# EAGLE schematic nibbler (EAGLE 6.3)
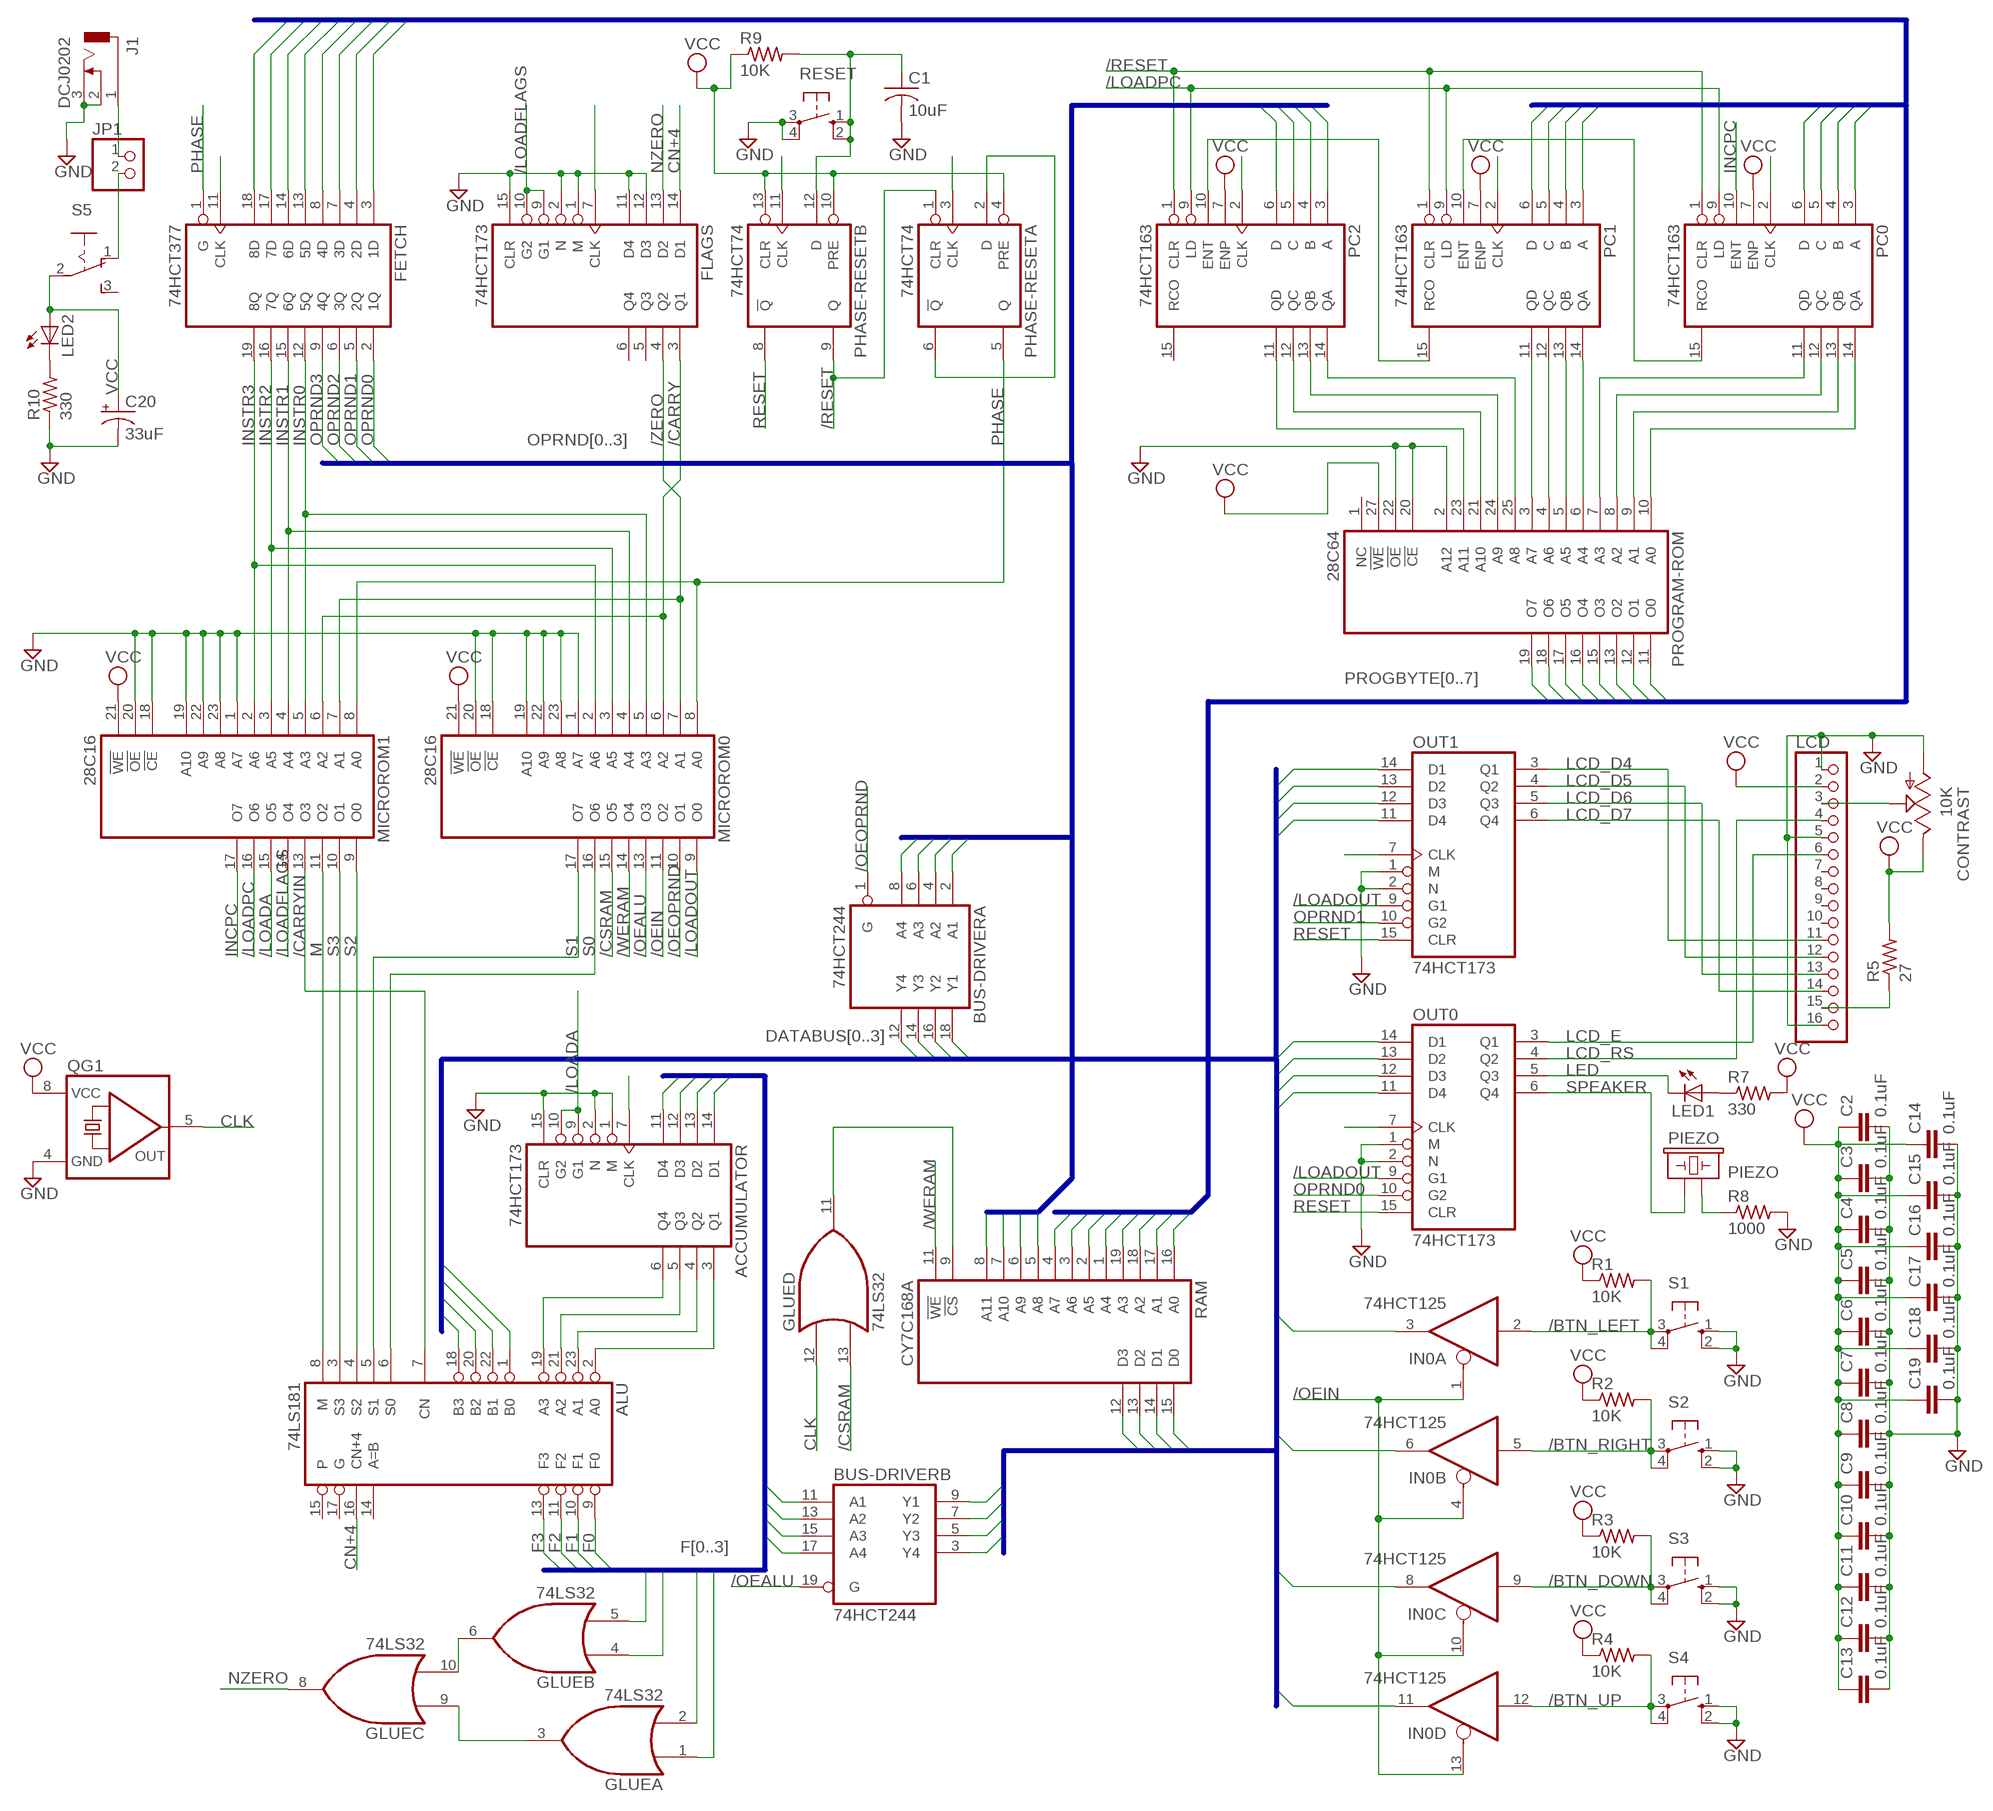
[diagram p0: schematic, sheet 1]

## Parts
ACCUMULATOR  74HCT173  74LS173N  [DIL16]
ALU  74LS181  74LS181N  [DIL24-6]
BUS-DRIVER  74HCT244  74LS244N  [DIL20]
C1  10uF  C-US025-024X044  [C025-024X044]
C2  0.1uF  C2,5-3  [C2.5-3]
C3  0.1uF  C2,5-3  [C2.5-3]
C4  0.1uF  C2,5-3  [C2.5-3]
C5  0.1uF  C2,5-3  [C2.5-3]
C6  0.1uF  C2,5-3  [C2.5-3]
C7  0.1uF  C2,5-3  [C2.5-3]
C8  0.1uF  C2,5-3  [C2.5-3]
C9  0.1uF  C2,5-3  [C2.5-3]
C10  0.1uF  C2,5-3  [C2.5-3]
C11  0.1uF  C2,5-3  [C2.5-3]
C12  0.1uF  C2,5-3  [C2.5-3]
C13  0.1uF  C2,5-3  [C2.5-3]
C14  0.1uF  C2,5-3  [C2.5-3]
C15  0.1uF  C2,5-3  [C2.5-3]
C16  0.1uF  C2,5-3  [C2.5-3]
C17  0.1uF  C2,5-3  [C2.5-3]
C18  0.1uF  C2,5-3  [C2.5-3]
C19  0.1uF  C2,5-3  [C2.5-3]
C20  33uF  CPOL-USTT5D10  [TT5D10]
CONTRAST  10K  TRIM_US-B25P  [B25P]
FETCH  74HCT377  74LS377N  [DIL20]
FLAGS  74HCT173  74LS173N  [DIL16]
GLUE  74LS32  74*32N  [DIL14]
IN0  74HCT125  74125N  [DIL14]
J1  DCJ0202  [DCJ0202]
JP1  PINHD-1X2  [1X02]
LCD  PINHD-1X16  [1X16]
LED1  LED5MM  [LED5MM]
LED2  LED5MM  [LED5MM]
MICROROM0  28C16  [DIL24]
MICROROM1  28C16  [DIL24]
OUT0  74HCT173  74LS173N  [DIL16]
OUT1  74HCT173  74LS173N  [DIL16]
PC0  74HCT163  74163N  [DIL16]
PC1  74HCT163  74163N  [DIL16]
PC2  74HCT163  74163N  [DIL16]
PHASE-RESET  74HCT74  74LS74N  [DIL14]
PIEZO  PIEZO  [PIEZO-12.6MM]
PROGRAM-ROM  28C64  [DIL28]
QG1  QG5460  [DIL08S]
R1  10K  R-US_0204/5  [0204/5]
R2  10K  R-US_0204/5  [0204/5]
R3  10K  R-US_0204/5  [0204/5]
R4  10K  R-US_0204/5  [0204/5]
R5  27  R-US_0204/5  [0204/5]
R7  330  R-US_0204/5  [0204/5]
R8  1000  R-US_0204/5  [0204/5]
R9  10K  R-US_0204/5  [0204/5]
R10  330  R-US_0204/5  [0204/5]
RAM  CY7C168A  51C68  [DIL20]
RESET  10-XX  [B3F-10XX]
S1  10-XX  [B3F-10XX]
S2  10-XX  [B3F-10XX]
S3  10-XX  [B3F-10XX]
S4  10-XX  [B3F-10XX]
S5  255SB  [255SB]

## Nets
/BTN_DOWN: IN0.9(C:I) R3.2 S3.3(P) S3.4(P1)
/BTN_LEFT: IN0.2(A:I) R1.2 S1.3(P) S1.4(P1)
/BTN_RIGHT: IN0.5(B:I) R2.2 S2.3(P) S2.4(P1)
/BTN_UP: IN0.12(D:I) R4.2 S4.3(P) S4.4(P1)
/CARRY: FLAGS.3(Q1) MICROROM0.6(A2) MICROROM1.6(A2)
/CARRYIN: ALU.7(CN) MICROROM1.13(O3)
/CSRAM: GLUE.13(D:I1) MICROROM0.15(O5)
/LOADA: ACCUMULATOR.9(G1) ACCUMULATOR.10(G2) MICROROM1.15(O5)
/LOADFLAGS: FLAGS.9(G1) FLAGS.10(G2) MICROROM1.14(O4)
/LOADOUT: MICROROM0.9(O0) OUT0.9(G1) OUT1.9(G1)
/LOADPC: MICROROM1.16(O6) PC0.9(LD) PC1.9(LD) PC2.9(LD)
/OEALU: BUS-DRIVER.19(B:G) MICROROM0.13(O3)
/OEIN: IN0.1(A:OE) IN0.4(B:OE) IN0.10(C:OE) IN0.13(D:OE) MICROROM0.11(O2)
/OEOPRND: BUS-DRIVER.1(A:G) MICROROM0.10(O1)
/RESET: PC0.1(CLR) PC1.1(CLR) PC2.1(CLR) PHASE-RESET.1(A:CLR) PHASE-RESET.9(B:Q)
/WERAM: MICROROM0.14(O4) RAM.11(!WE)
/ZERO: FLAGS.4(Q2) MICROROM0.7(A1) MICROROM1.7(A1)
CLK: ACCUMULATOR.7(CLK) FETCH.11(CLK) FLAGS.7(CLK) GLUE.12(D:I0) OUT0.7(CLK) OUT1.7(CLK) PC0.2(CLK) PC1.2(CLK) PC2.2(CLK) PHASE-RESET.3(A:CLK) PHASE-RESET.11(B:CLK) QG1.5(OUT)
CN+4: ALU.16(CN+4) FLAGS.14(D1)
DATABUS0: ALU.1(B0) BUS-DRIVER.9(B:Y1) BUS-DRIVER.18(A:Y1) IN0.3(A:O) OUT0.14(D1) OUT1.14(D1) RAM.15(D0)
DATABUS1: ALU.22(B1) BUS-DRIVER.7(B:Y2) BUS-DRIVER.16(A:Y2) IN0.6(B:O) OUT0.13(D2) OUT1.13(D2) RAM.14(D1)
DATABUS2: ALU.20(B2) BUS-DRIVER.5(B:Y3) BUS-DRIVER.14(A:Y3) IN0.8(C:O) OUT0.12(D3) OUT1.12(D3) RAM.13(D2)
DATABUS3: ALU.18(B3) BUS-DRIVER.3(B:Y4) BUS-DRIVER.12(A:Y4) IN0.11(D:O) OUT0.11(D4) OUT1.11(D4) RAM.12(D3)
F0: ACCUMULATOR.14(D1) ALU.9(F0) BUS-DRIVER.11(B:A1) GLUE.1(A:I0)
F1: ACCUMULATOR.13(D2) ALU.10(F1) BUS-DRIVER.13(B:A2) GLUE.2(A:I1)
F2: ACCUMULATOR.12(D3) ALU.11(F2) BUS-DRIVER.15(B:A3) GLUE.4(B:I0)
F3: ACCUMULATOR.11(D4) ALU.13(F3) BUS-DRIVER.17(B:A4) GLUE.5(B:I1)
GND: ACCUMULATOR.1(M) ACCUMULATOR.2(N) ACCUMULATOR.15(CLR) C1.2 C2.2 C3.2 C4.2 C5.2 C6.2 C7.2 C8.2 C9.2 C10.2 C11.2 C12.2 C13.2 C14.2 C15.2 C16.2 C17.2 C18.2 C19.2 C20.- CONTRAST.A FLAGS.1(M) FLAGS.2(N) FLAGS.11(D4) FLAGS.12(D3) FLAGS.15(CLR) J1.2 J1.3 LCD.1 LCD.5 LCD.16 MICROROM0.1(A7) MICROROM0.18(!CE) MICROROM0.19(A10) MICROROM0.20(!OE) MICROROM0.22(A9) MICROROM0.23(A8) MICROROM1.1(A7) MICROROM1.18(!CE) MICROROM1.19(A10) MICROROM1.20(!OE) MICROROM1.22(A9) MICROROM1.23(A8) OUT0.1(M) OUT0.2(N) OUT1.1(M) OUT1.2(N) PROGRAM-ROM.2(A12) PROGRAM-ROM.20(!CE) PROGRAM-ROM.22(!OE) QG1.4(GND) R8.2 R10.1 RESET.3(P) RESET.4(P1) S1.1(S) S1.2(S1) S2.1(S) S2.2(S1) S3.1(S) S3.2(S1) S4.1(S) S4.2(S1)
INCPC: MICROROM1.17(O7) PC0.10(ENT)
INSTR0: FETCH.12(5Q) MICROROM0.5(A3) MICROROM1.5(A3)
INSTR1: FETCH.15(6Q) MICROROM0.4(A4) MICROROM1.4(A4)
INSTR2: FETCH.16(7Q) MICROROM0.3(A5) MICROROM1.3(A5)
INSTR3: FETCH.19(8Q) MICROROM0.2(A6) MICROROM1.2(A6)
LCD_D4: LCD.11 OUT1.3(Q1)
LCD_D5: LCD.12 OUT1.4(Q2)
LCD_D6: LCD.13 OUT1.5(Q3)
LCD_D7: LCD.14 OUT1.6(Q4)
LCD_E: LCD.6 OUT0.3(Q1)
LCD_RS: LCD.4 OUT0.4(Q2)
LED: LED1.K(C) OUT0.5(Q3)
M: ALU.8(M) MICROROM1.11(O2)
N$1: PHASE-RESET.2(A:D) PHASE-RESET.6(A:!Q)
N$2: ACCUMULATOR.3(Q1) ALU.2(A0)
N$3: PC0.15(RCO) PC1.10(ENT)
N$4: ACCUMULATOR.4(Q2) ALU.23(A1)
N$5: ACCUMULATOR.5(Q3) ALU.21(A2)
N$6: ACCUMULATOR.6(Q4) ALU.19(A3)
N$7: PC1.15(RCO) PC2.10(ENT)
N$8: PC1.13(QB) PROGRAM-ROM.5(A5)
N$9: PC1.14(QA) PROGRAM-ROM.6(A4)
N$10: PC0.11(QD) PROGRAM-ROM.7(A3)
N$11: PC0.12(QC) PROGRAM-ROM.8(A2)
N$12: PC0.13(QB) PROGRAM-ROM.9(A1)
N$13: PC0.14(QA) PROGRAM-ROM.10(A0)
N$14: PC1.12(QC) PROGRAM-ROM.4(A6)
N$15: PC1.11(QD) PROGRAM-ROM.3(A7)
N$16: PC2.14(QA) PROGRAM-ROM.25(A8)
N$17: PC2.13(QB) PROGRAM-ROM.24(A9)
N$18: PC2.12(QC) PROGRAM-ROM.21(A10)
N$19: PC2.11(QD) PROGRAM-ROM.23(A11)
N$20: CONTRAST.S LCD.3
N$21: LCD.15 R5.1
N$22: LED1.A R7.1
N$23: PIEZO.- R8.1
N$24: C1.1 PHASE-RESET.12(B:D) R9.2 RESET.1(S) RESET.2(S1)
N$25: JP1.2 S5.1(O)
N$26: LED2.K(C) R10.2
N$27: GLUE.6(B:O) GLUE.10(C:I1)
N$28: J1.1 JP1.1
N$29: GLUE.3(A:O) GLUE.9(C:I0)
N$30: GLUE.11(D:O) RAM.9(!CS)
NZERO: FLAGS.13(D2) GLUE.8(C:O)
OPRND0: BUS-DRIVER.2(A:A1) FETCH.2(1Q) OUT0.10(G2) PC2.3(A) RAM.5(A8)
OPRND1: BUS-DRIVER.4(A:A2) FETCH.5(2Q) OUT1.10(G2) PC2.4(B) RAM.6(A9)
OPRND2: BUS-DRIVER.6(A:A3) FETCH.6(3Q) PC2.5(C) RAM.7(A10)
OPRND3: BUS-DRIVER.8(A:A4) FETCH.9(4Q) PC2.6(D) RAM.8(A11)
PHASE: FETCH.1(G) MICROROM0.8(A0) MICROROM1.8(A0) PHASE-RESET.5(A:Q)
PROGBYTE0: FETCH.3(1D) PC0.3(A) PROGRAM-ROM.11(O0) RAM.16(A0)
PROGBYTE1: FETCH.4(2D) PC0.4(B) PROGRAM-ROM.12(O1) RAM.17(A1)
PROGBYTE2: FETCH.7(3D) PC0.5(C) PROGRAM-ROM.13(O2) RAM.18(A2)
PROGBYTE3: FETCH.8(4D) PC0.6(D) PROGRAM-ROM.15(O3) RAM.19(A3)
PROGBYTE4: FETCH.13(5D) PC1.3(A) PROGRAM-ROM.16(O4) RAM.1(A4)
PROGBYTE5: FETCH.14(6D) PC1.4(B) PROGRAM-ROM.17(O5) RAM.2(A5)
PROGBYTE6: FETCH.17(7D) PC1.5(C) PROGRAM-ROM.18(O6) RAM.3(A6)
PROGBYTE7: FETCH.18(8D) PC1.6(D) PROGRAM-ROM.19(O7) RAM.4(A7)
RESET: OUT0.15(CLR) OUT1.15(CLR) PHASE-RESET.8(B:!Q)
S0: ALU.6(S0) MICROROM0.16(O6)
S1: ALU.5(S1) MICROROM0.17(O7)
S2: ALU.4(S2) MICROROM1.9(O0)
S3: ALU.3(S3) MICROROM1.10(O1)
SPEAKER: OUT0.6(Q4) PIEZO.+
VCC: C2.1 C3.1 C4.1 C5.1 C6.1 C7.1 C8.1 C9.1 C10.1 C11.1 C12.1 C13.1 C14.1 C15.1 C16.1 C17.1 C18.1 C19.1 C20.+ CONTRAST.E LCD.2 LED2.A MICROROM0.21(!WE) MICROROM1.21(!WE) PC0.7(ENP) PC1.7(ENP) PC2.7(ENP) PHASE-RESET.4(A:PRE) PHASE-RESET.10(B:PRE) PHASE-RESET.13(B:CLR) PROGRAM-ROM.27(!WE) QG1.8(VCC) R1.1 R2.1 R3.1 R4.1 R5.2 R7.2 R9.1 S5.2(P)
Unconnected: ALU.14(A=B) ALU.15(P) ALU.17(G) FLAGS.5(Q3) FLAGS.6(Q4) LCD.7 LCD.8 LCD.9 LCD.10 PC2.15(RCO) PROGRAM-ROM.1(NC) S5.3(S)

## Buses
OPRND[0..3]
DATABUS[0..3]
F[0..3]
PROGBYTE[0..7]

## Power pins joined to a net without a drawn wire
GND: ACCUMULATOR.8(GND) ALU.12(GND) BUS-DRIVER.10(P:GND) FETCH.10(GND) FLAGS.8(GND) GLUE.7(P:GND) IN0.7(P:GND) MICROROM0.12(GND) MICROROM1.12(GND) OUT0.8(GND) OUT1.8(GND) PC0.8(GND) PC1.8(GND) PC2.8(GND) PHASE-RESET.7(P:GND) PROGRAM-ROM.14(GND) RAM.10(GND)
VCC: ACCUMULATOR.16(VCC) ALU.24(VCC) BUS-DRIVER.20(P:VCC) FETCH.20(VCC) FLAGS.16(VCC) GLUE.14(P:VCC) IN0.14(P:VCC) MICROROM0.24(VCC) MICROROM1.24(VCC) OUT0.16(VCC) OUT1.16(VCC) PC0.16(VCC) PC1.16(VCC) PC2.16(VCC) PHASE-RESET.14(P:VCC) PROGRAM-ROM.28(VCC) RAM.20(VCC)

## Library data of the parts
ACCUMULATOR FLAGS OUT0 OUT1 = big-mess-o-wires:74*173: 4-bit D type REGISTER, 3-state
ALU = big-mess-o-wires:74*181: ARITHMETIC LOGIC UNIT function generator
BUS-DRIVER = big-mess-o-wires:74*244: Octal BUFFER and LINE DRIVER, 3-state
C1 = resistor:C-US: CAPACITOR, American symbol
C2-C19 = capacitor-wima:C: CAPACITOR
C20 = resistor:CPOL-US: POLARIZED CAPACITOR, American symbol
CONTRAST = pot:TRIM_US-: POTENTIOMETER
FETCH = big-mess-o-wires:74*377: Octal D type FLIP FLOP, enable
GLUE = big-mess-o-wires:74*32: Quad 2-input OR gate
IN0 = big-mess-o-wires:74*125: Quad bus BUFFER, 3-state
J1 = con-jack:DCJ0202: DC POWER JACK Source: DCJ0202.pdf; OC_FARNELL: unknown; OC_NEWARK: unknown
JP1 = pinhead:PINHD-1X2: PIN HEADER
LCD = pinhead:PINHD-1X16: PIN HEADER
LED1 LED2 = led:LED: LED
MICROROM0 MICROROM1 = big-mess-o-wires:28C16: MEMORY
PC0 PC1 PC2 = big-mess-o-wires:74*163: Synchronous 4-bit COUNTER
PHASE-RESET = big-mess-o-wires:74*74: Dual D type positive edge triggered FLIP FLOP, preset and clear
PIEZO = big-mess-o-wires:PIEZO: Piezo sounder
PROGRAM-ROM = big-mess-o-wires:28C64: MEMORY
QG1 = crystal:QG5460: CRYSTAL RESONATOR; OC_FARNELL: unknown; OC_NEWARK: unknown
R1-R5 R7-R10 = rcl:R-US_: RESISTOR, American symbol
RAM = memory:51C68: MEMORY
RESET S1-S4 = switch-omron:10-XX: OMRON SWITCH; MPN: B3F-1000; OC_FARNELL: 176432; OC_NEWARK: 36M3542
S5 = switch:255SB: SLIDING SWITCH Distributor Buerklin, 11G810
